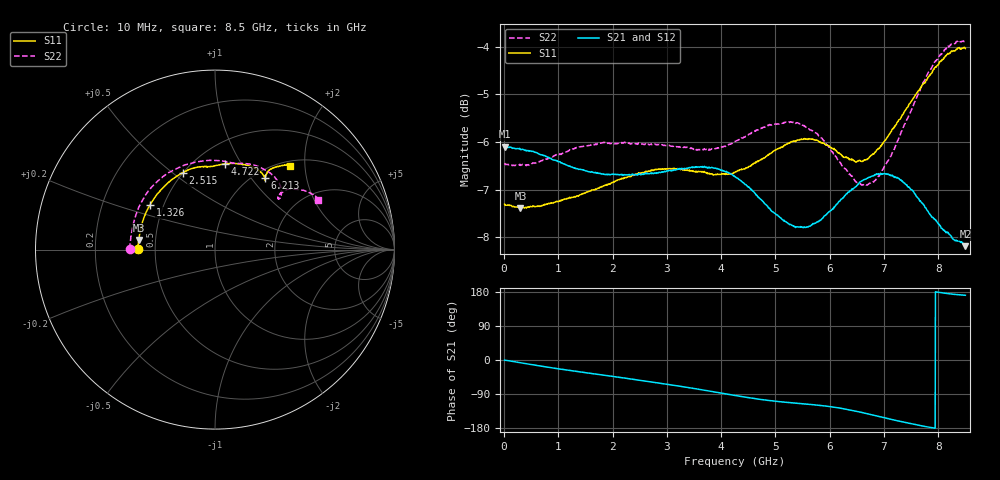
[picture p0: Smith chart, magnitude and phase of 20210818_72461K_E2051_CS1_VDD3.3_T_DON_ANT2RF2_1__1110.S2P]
!Agilent Technologies,E5071C,MY46417908,A.11.23
!Date: Wed Aug 18 14:27:01 2021
!Data & Calibration Information:
!Freq	S11:SOLT2(ON)	S21:SOLT2(ON)	S12:SOLT2(ON)	S22:SOLT2(ON)
!PortZ  Port1:50+j0  Port2:50+j0
!Above PortZ is port z conversion or system Z0 setting when saving the data.
!When reading, reference impedance value at option line is always used.
# Hz S dB R 50
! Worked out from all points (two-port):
!   1601 points, 10 MHz to 8.5 GHz, reference 50 ohm
!   highest |S21| = -6.10 dB at 10 MHz (marker M1); lowest = -8.2 dB at 8.5 GHz (marker M2)
!   |S21| within 3 dB of the highest: start of sweep to end of sweep
!   lowest |S11| = -7.4 dB at 301.8 MHz (marker M3), VSWR 2.49, Z = 20.1 + j2.61 ohm
!   |S11| at or under -10 dB: nowhere
!   |S22| runs from -6.9 to -3.9 dB; largest |S21 - S12| = 0.0018
!   S11 on the Smith chart (normalised r, x): 10 MHz: 0.40, +0.00; 1.326 GHz: 0.42, +0.26; 2.515 GHz: 0.50, +0.54; 4.722 GHz: 0.68, +0.85; 6.213 GHz: 1.12, +1.17; 8.5 GHz: 1.09, +1.68
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1e7  -7.31 179.6  -6.10 -0.4  -6.09 -0.4  -6.44 179.6
3.018438e8  -7.39 172.9  -6.16 -7.2  -6.14 -7.2  -6.49 170.9
8.961438e8  -7.28 157.9  -6.37 -21.0  -6.37 -21.0  -6.31 152.9
1.32595e9  -7.14 145.4  -6.56 -30.0  -6.56 -30.0  -6.12 139.0
1.426769e9  -7.10 142.3  -6.58 -32.0  -6.58 -32.0  -6.09 135.7
1.872494e9  -6.91 128.9  -6.68 -40.8  -6.69 -40.8  -6.01 121.2
2.51455e9  -6.65 112.9  -6.68 -53.6  -6.68 -53.7  -6.04 102.2
2.843538e9  -6.57 106.7  -6.64 -60.6  -6.64 -60.6  -6.06 94.1
3.241506e9  -6.57 101.0  -6.56 -69.3  -6.55 -69.4  -6.10 86.2
3.655394e9  -6.62 96.7  -6.52 -78.9  -6.51 -79.0  -6.15 80.2
4.255e9  -6.63 90.6  -6.73 -93.6  -6.72 -93.6  -5.99 73.1
4.72195e9  -6.38 83.6  -7.20 -103.9  -7.19 -103.9  -5.72 66.0
5.210125e9  -6.04 72.7  -7.69 -111.9  -7.70 -111.8  -5.58 55.8
5.671769e9  -5.94 62.5  -7.74 -117.7  -7.75 -117.6  -5.76 46.5
5.931775e9  -6.07 57.9  -7.53 -121.6  -7.56 -121.6  -6.04 42.4
6.213006e9  -6.26 55.3  -7.20 -127.5  -7.22 -127.6  -6.46 39.3
6.616281e9  -6.40 54.4  -6.80 -139.3  -6.81 -139.3  -6.90 38.5
7.088538e9  -5.85 55.8  -6.68 -155.3  -6.69 -155.3  -6.37 40.7
7.422831e9  -5.28 55.4  -6.91 -165.9  -6.91 -165.9  -5.52 39.5
7.8208e9  -4.63 52.4  -7.48 -177.0  -7.46 -177.1  -4.53 33.9
8.197544e9  -4.15 49.7  -7.93 174.8  -7.91 174.8  -4.00 28.5
8.5e9  -4.04 48.2  -8.19 170.7  -8.16 170.6  -3.92 25.8
